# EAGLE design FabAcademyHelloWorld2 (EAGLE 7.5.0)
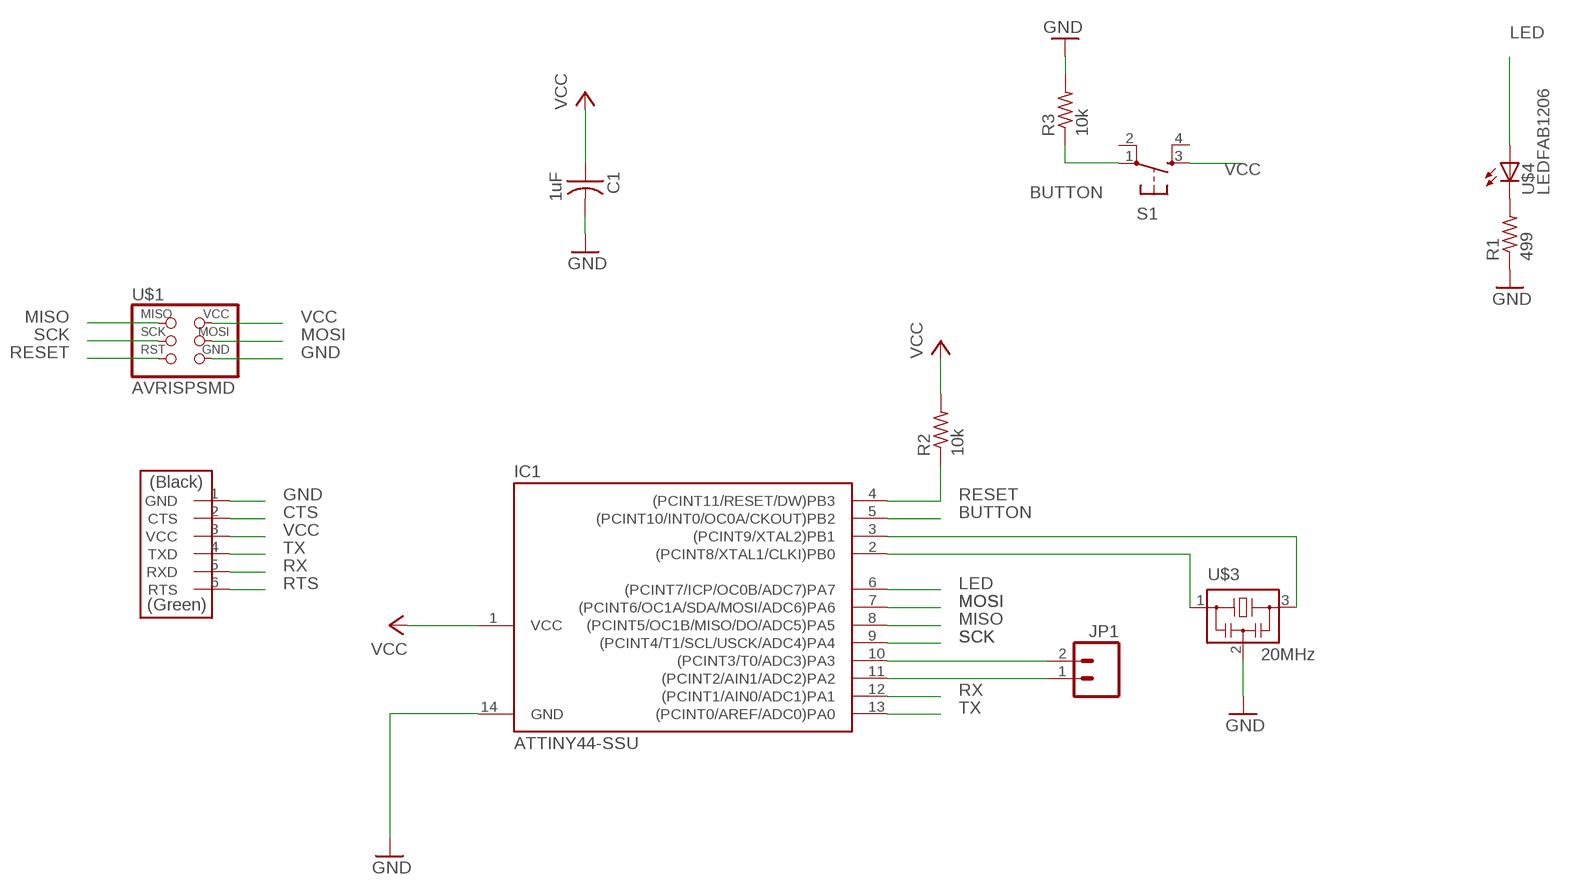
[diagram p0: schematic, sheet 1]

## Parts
C1  1uF  CAP-US1206FAB  [C1206FAB]
IC1  ATTINY44-SSU  [SOIC14]
JP1  M02PTH  [1X02]
R1  499  RES-US1206FAB  [R1206FAB]
R2  10k  RES-US1206FAB  [R1206FAB]
R3  10k  RES-US1206FAB  [R1206FAB]
S1  6MM_SWITCH6MM_SWITCH  [6MM_SWITCH]
U$1  AVRISPSMD  [2X03SMD]
U$2  FTDI-SMD-HEADER  [1X06SMD]
U$3  20MHz  RESONATOR  [EFOBM]
U$4  LEDFAB1206  [LED1206FAB]

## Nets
BUTTON: IC1.5((PCINT10/INT0/OC0A/CKOUT)PB2) R3.1 S1.1(P)
CTS: U$2.2(CTS)
GND: C1.2 IC1.14(GND) R1.1 R3.2 U$1.6(GND) U$2.1(GND) U$3.2
LED: IC1.6((PCINT7/ICP/OC0B/ADC7)PA7) U$4.1(A)
MISO: IC1.8((PCINT5/OC1B/MISO/DO/ADC5)PA5) U$1.1(MISO)
MOSI: IC1.7((PCINT6/OC1A/SDA/MOSI/ADC6)PA6) U$1.4(MOSI)
N$1: R1.2 U$4.2(C)
N$2: IC1.2((PCINT8/XTAL1/CLKI)PB0) U$3.1
N$3: IC1.11((PCINT2/AIN1/ADC2)PA2) JP1.1
N$4: IC1.10((PCINT3/T0/ADC3)PA3) JP1.2
N$9: IC1.3((PCINT9/XTAL2)PB1) U$3.3
RESET: IC1.4((PCINT11/RESET/DW)PB3) R2.1 U$1.5(RST)
RTS: U$2.6(RTS)
RX: IC1.12((PCINT1/AIN0/ADC1)PA1) U$2.5(RXD)
SCK: IC1.9((PCINT4/T1/SCL/USCK/ADC4)PA4) U$1.3(SCK)
TX: IC1.13((PCINT0/AREF/ADC0)PA0) U$2.4(TXD)
VCC: C1.1 IC1.1(VCC) R2.2 S1.3(S) U$1.2(VCC) U$2.3(VCC)
Unconnected: S1.2(P1) S1.4(S1)

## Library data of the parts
C1 = fablab:CAP-US
IC1 = fablab:ATTINY44
JP1 = SparkFun-Connectors:M02: Standard 2-pin 0.1" header. Use with
R1-R3 = fablab:RES-US: Resistor (US Symbol)
S1 = fablab:6MM_SWITCH: OMRON SWITCH
U$1 = fablab:AVRISP
U$2 = fablab:FTDI-SMD-HEADER
U$3 = fablab:RESONATOR
U$4 = fablab:LED: LED

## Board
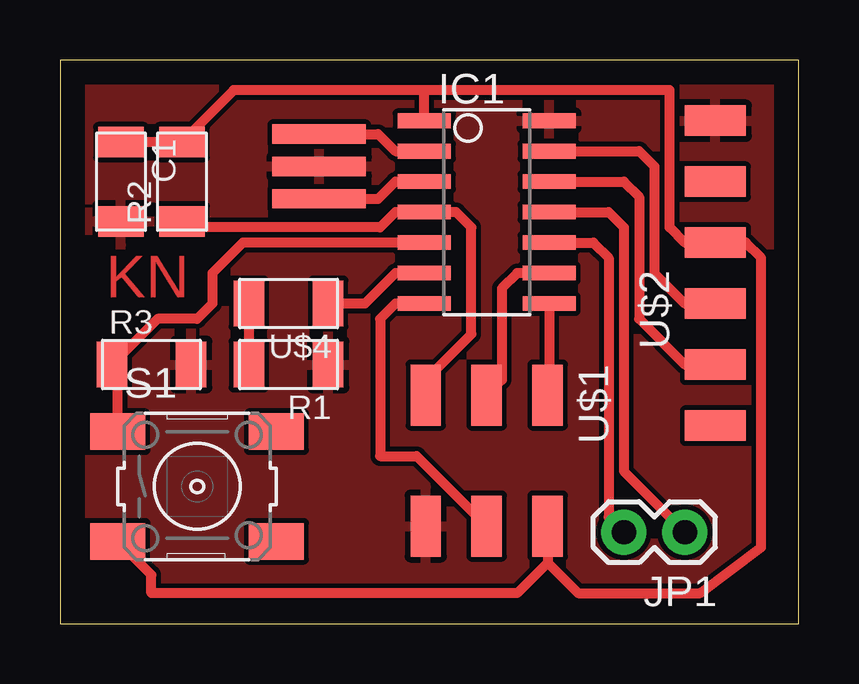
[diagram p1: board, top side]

Size 30.79 x 23.48 mm. Coordinates in mm from the lower left corner, seen from the top.
Outline: 0,0 30.79,0 30.79,23.48 0,23.48 0,0
Copper layers (1*16): Top 0.035mm / dielectric 1.5mm / Bottom 0.035mm
Design rules "default *": minimum track width 16mil, minimum drill 24mil, track to track 8mil, track to pad 8mil, pad to pad 8mil, via to via 8mil, smd to smd 8mil, copper to edge 40mil, drill to drill 8mil, minimum pad ring 10mil, minimum via ring 8mil, stop-mask expansion 4mil, vias tented up to drill 0mil, thermal gap 10mil

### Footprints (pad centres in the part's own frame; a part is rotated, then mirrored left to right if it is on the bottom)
C1206FAB = smd 1.27 x 1.905: 1 -1.651,0; 2 1.651,0
SOIC14 = smd 0.61 x 2.21: 1 -3.81,-2.603; 2 -2.54,-2.603; 3 -1.27,-2.603; 4 0,-2.603; 5 1.27,-2.603; 6 2.54,-2.603; 7 3.81,-2.603; 8 3.81,2.603; 9 2.54,2.603; 10 1.27,2.603; 11 0,2.603; 12 -1.27,2.603; 13 -2.54,2.603; 14 -3.81,2.603
1X02 = drill 1.016 pad 1.88: 1 0,0; 2 2.54,0
R1206FAB = smd 1.27 x 1.905: 1 -1.651,0; 2 1.651,0
6MM_SWITCH = smd 2.286 x 1.524: 1 -3.302,2.286; 2 3.302,2.286; 3 -3.302,-2.286; 4 3.302,-2.286
2X03SMD = smd 2.54 x 1.27: 1 -2.54,2.54; 2 2.92,2.54; 3 -2.54,0; 4 2.92,0; 5 -2.54,-2.54; 6 2.92,-2.54
1X06SMD = smd 2.54 x 1.27: 1 0,6.35; 2 0,3.81; 3 0,1.27; 4 0,-1.27; 5 0,-3.81; 6 0,-6.35
EFOBM = smd 0.8 x 3.9: 1 -1.35,0; 2 0,0; 3 1.35,0
LED1206FAB = smd 1.27 x 1.905: 1 -1.651,0; 2 1.651,0

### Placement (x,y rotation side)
C1  2.54,18.41 270 top
IC1  17.78,17.14 270 top
JP1  26.04,3.81 180 top
R1  9.52,10.8 180 top
R2  5.08,18.41 90 top
R3  3.81,10.8 0 top
S1  5.71,5.71 0 top
U$1  17.78,6.98 270 top
U$2  27.3,14.6 0 top
U$3  10.79,19.05 270 top
U$4  9.52,13.34 180 top

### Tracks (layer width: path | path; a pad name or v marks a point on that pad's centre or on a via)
BUTTON
  Top 0.406: S1.1 2.41,10.54 R3.1 4.06,12.7 5.71,12.7 6.35,13.34 6.35,14.6 7.62,15.88 IC1.5
GND
  pour Top: 0.63,22.86 29.85,22.86 29.85,0.63 0.63,0.63
LED
  Top 0.406: IC1.6 13.97,14.6 12.7,13.34 U$4.1
MISO
  Top 0.406: IC1.8 20.38,9.59 U$1.1
MOSI
  Top 0.406: IC1.7 13.97,13.34 13.33,12.7 13.33,6.98 14.86,6.98 U$1.4
N$1
  Top 0.406: U$4.2 R1.2
N$2
  Top 0.406: U$3.1 13.25,20.4 13.97,19.69 IC1.2
N$3
  Top 0.406: IC1.11 22.86,17.14 23.5,16.51 23.5,6.35 JP1.1
N$4
  Top 0.406: IC1.10 22.22,15.88 22.86,15.24 22.86,4.45 JP1.2
N$9
  Top 0.406: U$3.3 13.25,17.7 13.97,18.41 IC1.3
RESET
  Top 0.406: R2.1 5.33,16.51 13.33,16.51 13.97,17.14 IC1.4 16.51,17.14 17.14,16.51 17.14,12.06 15.24,10.16 U$1.5
RX
  Top 0.406: IC1.12 23.5,18.41 24.13,17.78 24.13,12.7 26.04,10.8 U$2.5
SCK
  Top 0.406: IC1.9 19.05,14.6 18.42,13.97 18.42,10.16 U$1.3
TX
  Top 0.406: IC1.13 24.13,19.69 24.76,19.05 24.76,14.6 26.04,13.34 U$2.4
VCC
  Top 0.406: 20.32,2.54 19.05,1.27 3.81,1.27 3.81,2.03 S1.3 | 15.24,22.23 25.4,22.23 25.4,16.51 26.04,15.88 U$2.3 28.57,15.88 29.21,15.24 29.21,3.18 26.67,1.27 21.59,1.27 20.32,2.54 | 15.24,22.23 7.24,22.23 R2.2 C1.1 | IC1.1 15.18,22.16 15.24,22.23 | U$1.2 20.32,2.54

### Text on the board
Top: KN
